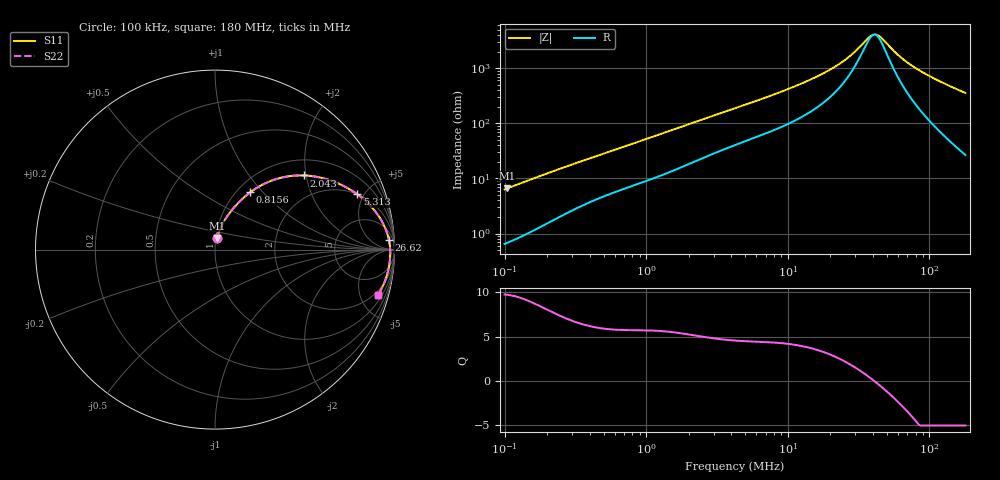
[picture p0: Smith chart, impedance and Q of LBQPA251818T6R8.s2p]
! LBQPA251818T6R8  S-PARAMETER MODEL  ( General Type )
! Model Generated by TAIYO YUDEN Corporation (http://www.ty-top.com)
! Version 1.0
! TAIYO YUDEN Control No. 191025NI43SB-FBB
! Copyright(c) 2019 TAIYO YUDEN CO.,LTD. All Rights Reserved.
! Product Description (link to TY-COMPAS)
! https://ds.yuden.co.jp/TYCOMPAS/or/detail?pn=LBQPA251818T6R8M&u=M
! Products Name : Inductors
! Characteristics :
!  Inductance : 6.8 uH , SRF(min) : 38 MHz , DC Resistance(max) : 0.39 Ohm
!  Rated Current : Saturation :550 mA , Temp Rise : 420 mA (20 degC)
!  Case Size : 2.5 x 1.8 / 0.098 x 0.071 [mm/inch] , Thickness : 1.8 / 0.071 [mm/inch]
!  (Conditions: Temperature = 25 degC , DC Bias Current/Voltage = 0A / 0V)
! External Node Assignments :
!  1  o---GGG---o  2
! GND o---------o GND
! Frequency Range : 0.1MHz  -  180.004543MHz  [ 402 STEP ]
# MHz S RI R 50
! Freq[MHz].  S11 Real  S11 Imag  S21 Real  S21 Imag  S12 Real  S12 Imag  S22 Real  S22 Imag
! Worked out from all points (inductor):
!   401 points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, 100 kHz to 180 MHz, reference 50 ohm
!   read as one part in series: L = 9.96 uH near 103.8 kHz
!   highest Q = 9.7 at 103.8 kHz (marker M1), where L = 10 uH
!   self-resonance near 40.89 MHz
!   S11 on the Smith chart (normalised r, x): 100 kHz: 1.01, +0.13; 815.6 kHz: 1.15, +0.85; 2.043 MHz: 1.37, +1.94; 5.313 MHz: 2.00, +4.46; 26.62 MHz: 15, +28; 180 MHz: 1.53, -7.08
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0.1  0.0103 0.062  0.9897 -0.062  0.9897 -0.062  0.0103 0.062
0.103819  0.0109 0.0643  0.9891 -0.0643  0.9891 -0.0643  0.0109 0.0643
0.350962  0.0672 0.1842  0.9328 -0.1842  0.9328 -0.1842  0.0672 0.1842
0.550271  0.1214 0.2518  0.8786 -0.2518  0.8786 -0.2518  0.1214 0.2518
0.815604  0.1957 0.3188  0.8043 -0.3188  0.8043 -0.3188  0.1957 0.3188
1.231743  0.3111 0.3826  0.6889 -0.3826  0.6889 -0.3826  0.3111 0.3826
2.042921  0.4947 0.4131  0.5053 -0.4131  0.5053 -0.4131  0.4947 0.4131
2.86246  0.6165 0.3939  0.3835 -0.3939  0.3835 -0.3939  0.6165 0.3939
4.322947  0.7415 0.3413  0.2585 -0.3413  0.2585 -0.3413  0.7415 0.3413
5.312516  0.7926 0.3086  0.2074 -0.3086  0.2074 -0.3086  0.7926 0.3086
9.147624  0.8912 0.2152  0.1088 -0.2152  0.1088 -0.2152  0.8912 0.2152
14.89024  0.941 0.1358  0.059 -0.1358  0.059 -0.1358  0.941 0.1358
20.47629  0.9594 0.0896  0.0406 -0.0896  0.0406 -0.0896  0.9594 0.0896
26.61866  0.9689 0.0545  0.0311 -0.0545  0.0311 -0.0545  0.9689 0.0545
37.297  0.9753 0.0116  0.0247 -0.0116  0.0247 -0.0116  0.9753 0.0116
40.20007  0.976 0.00215  0.024 -0.00215  0.024 -0.00215  0.976 0.00215
44.14869  0.9765 -0.00973  0.0235 0.00973  0.0235 0.00973  0.9765 -0.00973
52.25907  0.9764 -0.0315  0.0236 0.0315  0.0236 0.0315  0.9764 -0.0315
65.43652  0.9743 -0.0622  0.0257 0.0622  0.0257 0.0622  0.9743 -0.0622
85.06583  0.9682 -0.1017  0.0318 0.1017  0.0318 0.1017  0.9682 -0.1017
121.4454  0.9507 -0.1647  0.0493 0.1647  0.0493 0.1647  0.9507 -0.1647
180.0045  0.9105 -0.2504  0.0895 0.2504  0.0895 0.2504  0.9105 -0.2504
